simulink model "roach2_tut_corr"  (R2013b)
settings: Solver=VariableStepDiscrete  SolverMode=SingleTasking  StartTime=0.0  StopTime=100  RelTol=1e-3
undefined symbols (not defined in the file): add_latency, addr_width, Bit, bitfield, BitWidth, bram_latency, burst_size, casper_library_scopes, conv_latency, data_width, DelayLen, fan_latency, FFTSize, FFTStage, getfield, increment, led, Location, Lower, mult_latency, mux_latency, n_bits, n_bits_data, n_inputs, n_streams, n_taps, neg_latency, negate_latency, nsamples, pfb_size, pulse_len, reset_period, ROACH, ROACH2, snapshot, sx475t, sync_period, sync_period_bits, Upper, UseCounter, Width
libraries: xbsIndex_r4 x24444, casper_library_misc x73, xbsReplacements_r4 x34, casper_library_delays x14, xps_library x7
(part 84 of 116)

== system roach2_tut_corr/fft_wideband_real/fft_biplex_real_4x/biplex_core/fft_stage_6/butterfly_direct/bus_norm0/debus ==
  bus_in : Inport
  reinterpret{1..16} (16 alike) : xbsIndex_r4/Reinterpret  force_arith_type=on  arith_type="Signed  (2's comp)"  force_bin_pt=on  bin_pt=17  block_type=reinterpret
  slice1 : xbsIndex_r4/Slice  nbits=20  boolean_output=off  mode=Upper Bit Location + Width  bit1=-300  base1=MSB of Input  bit0=0  base0=LSB of Input  dbl_ovrd=off  block_type=slice
  slice10 : xbsIndex_r4/Slice  nbits=20  boolean_output=off  mode=Upper Bit Location + Width  bit1=-120  base1=MSB of Input  bit0=0  base0=LSB of Input  dbl_ovrd=off  block_type=slice
  slice11 : xbsIndex_r4/Slice  nbits=20  boolean_output=off  mode=Upper Bit Location + Width  bit1=-100  base1=MSB of Input  bit0=0  base0=LSB of Input  dbl_ovrd=off  block_type=slice
  slice12 : xbsIndex_r4/Slice  nbits=20  boolean_output=off  mode=Upper Bit Location + Width  bit1=-80  base1=MSB of Input  bit0=0  base0=LSB of Input  dbl_ovrd=off  block_type=slice
  slice13 : xbsIndex_r4/Slice  nbits=20  boolean_output=off  mode=Upper Bit Location + Width  bit1=-60  base1=MSB of Input  bit0=0  base0=LSB of Input  dbl_ovrd=off  block_type=slice
  slice14 : xbsIndex_r4/Slice  nbits=20  boolean_output=off  mode=Upper Bit Location + Width  bit1=-40  base1=MSB of Input  bit0=0  base0=LSB of Input  dbl_ovrd=off  block_type=slice
  slice15 : xbsIndex_r4/Slice  nbits=20  boolean_output=off  mode=Upper Bit Location + Width  bit1=-20  base1=MSB of Input  bit0=0  base0=LSB of Input  dbl_ovrd=off  block_type=slice
  slice16 : xbsIndex_r4/Slice  nbits=20  boolean_output=off  mode=Upper Bit Location + Width  bit1=0  base1=MSB of Input  bit0=0  base0=LSB of Input  dbl_ovrd=off  block_type=slice
  slice2 : xbsIndex_r4/Slice  nbits=20  boolean_output=off  mode=Upper Bit Location + Width  bit1=-280  base1=MSB of Input  bit0=0  base0=LSB of Input  dbl_ovrd=off  block_type=slice
  slice3 : xbsIndex_r4/Slice  nbits=20  boolean_output=off  mode=Upper Bit Location + Width  bit1=-260  base1=MSB of Input  bit0=0  base0=LSB of Input  dbl_ovrd=off  block_type=slice
  slice4 : xbsIndex_r4/Slice  nbits=20  boolean_output=off  mode=Upper Bit Location + Width  bit1=-240  base1=MSB of Input  bit0=0  base0=LSB of Input  dbl_ovrd=off  block_type=slice
  slice5 : xbsIndex_r4/Slice  nbits=20  boolean_output=off  mode=Upper Bit Location + Width  bit1=-220  base1=MSB of Input  bit0=0  base0=LSB of Input  dbl_ovrd=off  block_type=slice
  slice6 : xbsIndex_r4/Slice  nbits=20  boolean_output=off  mode=Upper Bit Location + Width  bit1=-200  base1=MSB of Input  bit0=0  base0=LSB of Input  dbl_ovrd=off  block_type=slice
  slice7 : xbsIndex_r4/Slice  nbits=20  boolean_output=off  mode=Upper Bit Location + Width  bit1=-180  base1=MSB of Input  bit0=0  base0=LSB of Input  dbl_ovrd=off  block_type=slice
  slice8 : xbsIndex_r4/Slice  nbits=20  boolean_output=off  mode=Upper Bit Location + Width  bit1=-160  base1=MSB of Input  bit0=0  base0=LSB of Input  dbl_ovrd=off  block_type=slice
  slice9 : xbsIndex_r4/Slice  nbits=20  boolean_output=off  mode=Upper Bit Location + Width  bit1=-140  base1=MSB of Input  bit0=0  base0=LSB of Input  dbl_ovrd=off  block_type=slice
  msb_out16 : Outport
  out15 : Outport  Port=2
  out14 : Outport  Port=3
  out13 : Outport  Port=4
  out12 : Outport  Port=5
  out11 : Outport  Port=6
  out10 : Outport  Port=7
  out9 : Outport  Port=8
  out8 : Outport  Port=9
  out7 : Outport  Port=10
  out6 : Outport  Port=11
  out5 : Outport  Port=12
  out4 : Outport  Port=13
  out3 : Outport  Port=14
  out2 : Outport  Port=15
  lsb_out1 : Outport  Port=16
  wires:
  bus_in/1 -> slice16/1, slice15/1, slice14/1, slice13/1, slice12/1, slice11/1, slice10/1, slice9/1, slice8/1, slice7/1, slice6/1, slice5/1, slice4/1, slice3/1, slice2/1, slice1/1
  slice16/1 -> reinterpret16/1
  reinterpret16/1 -> msb_out16/1
  slice15/1 -> reinterpret15/1
  reinterpret15/1 -> out15/1
  slice14/1 -> reinterpret14/1
  reinterpret14/1 -> out14/1
  slice13/1 -> reinterpret13/1
  reinterpret13/1 -> out13/1
  slice12/1 -> reinterpret12/1
  reinterpret12/1 -> out12/1
  slice11/1 -> reinterpret11/1
  reinterpret11/1 -> out11/1
  slice10/1 -> reinterpret10/1
  reinterpret10/1 -> out10/1
  slice9/1 -> reinterpret9/1
  reinterpret9/1 -> out9/1
  slice8/1 -> reinterpret8/1
  reinterpret8/1 -> out8/1
  slice7/1 -> reinterpret7/1
  reinterpret7/1 -> out7/1
  slice6/1 -> reinterpret6/1
  reinterpret6/1 -> out6/1
  slice5/1 -> reinterpret5/1
  reinterpret5/1 -> out5/1
  slice4/1 -> reinterpret4/1
  reinterpret4/1 -> out4/1
  slice3/1 -> reinterpret3/1
  reinterpret3/1 -> out3/1
  slice2/1 -> reinterpret2/1
  reinterpret2/1 -> out2/1
  slice1/1 -> reinterpret1/1
  reinterpret1/1 -> lsb_out1/1

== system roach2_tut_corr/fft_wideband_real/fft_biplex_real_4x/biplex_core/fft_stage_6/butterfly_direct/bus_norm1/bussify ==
  in1 : Inport
  in2 : Inport  Port=2
  in3 : Inport  Port=3
  in4 : Inport  Port=4
  in5 : Inport  Port=5
  in6 : Inport  Port=6
  in7 : Inport  Port=7
  in8 : Inport  Port=8
  in9 : Inport  Port=9
  in10 : Inport  Port=10
  in11 : Inport  Port=11
  in12 : Inport  Port=12
  in13 : Inport  Port=13
  in14 : Inport  Port=14
  in15 : Inport  Port=15
  in16 : Inport  Port=16
  concatenate : xbsIndex_r4/Concat  num_inputs=16  dbl_ovrd=off  block_type=concat
  reinterpret{1..16} (16 alike) : xbsIndex_r4/Reinterpret  force_arith_type=on  arith_type=Unsigned  force_bin_pt=on  bin_pt=0  block_type=reinterpret
  bus_out : Outport
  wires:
  concatenate/1 -> bus_out/1
  in1/1 -> reinterpret1/1
  reinterpret1/1 -> concatenate/1
  in2/1 -> reinterpret2/1
  reinterpret2/1 -> concatenate/2
  in3/1 -> reinterpret3/1
  reinterpret3/1 -> concatenate/3
  in4/1 -> reinterpret4/1
  reinterpret4/1 -> concatenate/4
  in5/1 -> reinterpret5/1
  reinterpret5/1 -> concatenate/5
  in6/1 -> reinterpret6/1
  reinterpret6/1 -> concatenate/6
  in7/1 -> reinterpret7/1
  reinterpret7/1 -> concatenate/7
  in8/1 -> reinterpret8/1
  reinterpret8/1 -> concatenate/8
  in9/1 -> reinterpret9/1
  reinterpret9/1 -> concatenate/9
  in10/1 -> reinterpret10/1
  reinterpret10/1 -> concatenate/10
  in11/1 -> reinterpret11/1
  reinterpret11/1 -> concatenate/11
  in12/1 -> reinterpret12/1
  reinterpret12/1 -> concatenate/12
  in13/1 -> reinterpret13/1
  reinterpret13/1 -> concatenate/13
  in14/1 -> reinterpret14/1
  reinterpret14/1 -> concatenate/14
  in15/1 -> reinterpret15/1
  reinterpret15/1 -> concatenate/15
  in16/1 -> reinterpret16/1
  reinterpret16/1 -> concatenate/16

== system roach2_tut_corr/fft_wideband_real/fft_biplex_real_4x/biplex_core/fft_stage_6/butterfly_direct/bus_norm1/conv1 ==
  note: (ones_bit & 1) -> round-to-even (ones_bit ^ 1) -> round-to-odd (sign_bit & 1)-> round-to-zero (sign_bit ^ 1) -> round-to-inf (X ~| 1) -> round half down (X | 1) -> round half up
  in : Inport
  Concat : xbsIndex_r4/Concat  num_inputs=2  dbl_ovrd=off  block_type=concat
  Constant : xbsIndex_r4/Constant  const=1  gui_display_data_type=Fixed-point  arith_type=Unsigned  n_bits=1  bin_pt=0  preci_type=Single  exp_width=8  frac_width=24  explicit_period=off  period=1  equ=P=C  opselect=C  inp2=PCIN>>17  opr=+  inp1=P  carry=CIN  dbl_ovrd=off  block_type=constant
  Reinterpret : xbsIndex_r4/Reinterpret  force_arith_type=on  arith_type=Unsigned  force_bin_pt=on  bin_pt=0  block_type=reinterpret
  adder : xbsIndex_r4/AddSub  mode=Addition  use_carryin=off  use_carryout=off  en=off  latency=0  precision=User Defined  arith_type="Signed  (2's comp)"  n_bits=21  bin_pt=18  quantization=Truncate  overflow=Wrap  dbl_ovrd=off  use_behavioral_HDL=off  hw_selection=Fabric  pipelined=on  use_rpm=on  block_type=addsub
  almost_half : xbsIndex_r4/Constant  const=0  gui_display_data_type=Fixed-point  arith_type=Unsigned  n_bits=19  bin_pt=0  preci_type=Single  exp_width=8  frac_width=24  explicit_period=off  period=1  equ=P=C  opselect=C  inp2=PCIN>>17  opr=+  inp1=P  carry=CIN  dbl_ovrd=off  block_type=constant
  bit : xbsIndex_r4/Slice  nbits=1  boolean_output=off  mode=Lower Bit Location + Width  bit1=0  base1=MSB of Input  bit0=0  base0=LSB of Input  dbl_ovrd=off  block_type=slice
  force1 : xbsIndex_r4/Reinterpret  force_arith_type=on  arith_type="Signed  (2's comp)"  force_bin_pt=on  bin_pt=19  block_type=reinterpret
  force2 : xbsIndex_r4/Reinterpret  force_arith_type=off  arith_type="Signed  (2's comp)"  force_bin_pt=on  bin_pt=19  block_type=reinterpret
  tweak_op : xbsIndex_r4/Logical  logical_function=NOR  inputs=2  en=off  latency=0  precision=Full  arith_type=Unsigned  n_bits=8  bin_pt=2  align_bp=on  dbl_ovrd=off  block_type=logical
  out : Outport
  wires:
  tweak_op/1 -> Concat/2
  Constant/1 -> tweak_op/2
  bit/1 -> tweak_op/1
  almost_half/1 -> force2/1
  in/1 -> Reinterpret/1, bit/1
  Concat/1 -> force1/1
  Reinterpret/1 -> Concat/1
  force1/1 -> adder/1
  force2/1 -> adder/2
  adder/1 -> out/1

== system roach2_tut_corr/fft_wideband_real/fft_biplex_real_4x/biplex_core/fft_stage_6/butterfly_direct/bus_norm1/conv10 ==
  note: (ones_bit & 1) -> round-to-even (ones_bit ^ 1) -> round-to-odd (sign_bit & 1)-> round-to-zero (sign_bit ^ 1) -> round-to-inf (X ~| 1) -> round half down (X | 1) -> round half up
  in : Inport
  Concat : xbsIndex_r4/Concat  num_inputs=2  dbl_ovrd=off  block_type=concat
  Constant : xbsIndex_r4/Constant  const=1  gui_display_data_type=Fixed-point  arith_type=Unsigned  n_bits=1  bin_pt=0  preci_type=Single  exp_width=8  frac_width=24  explicit_period=off  period=1  equ=P=C  opselect=C  inp2=PCIN>>17  opr=+  inp1=P  carry=CIN  dbl_ovrd=off  block_type=constant
  Reinterpret : xbsIndex_r4/Reinterpret  force_arith_type=on  arith_type=Unsigned  force_bin_pt=on  bin_pt=0  block_type=reinterpret
  adder : xbsIndex_r4/AddSub  mode=Addition  use_carryin=off  use_carryout=off  en=off  latency=0  precision=User Defined  arith_type="Signed  (2's comp)"  n_bits=21  bin_pt=18  quantization=Truncate  overflow=Wrap  dbl_ovrd=off  use_behavioral_HDL=off  hw_selection=Fabric  pipelined=on  use_rpm=on  block_type=addsub
  almost_half : xbsIndex_r4/Constant  const=0  gui_display_data_type=Fixed-point  arith_type=Unsigned  n_bits=19  bin_pt=0  preci_type=Single  exp_width=8  frac_width=24  explicit_period=off  period=1  equ=P=C  opselect=C  inp2=PCIN>>17  opr=+  inp1=P  carry=CIN  dbl_ovrd=off  block_type=constant
  bit : xbsIndex_r4/Slice  nbits=1  boolean_output=off  mode=Lower Bit Location + Width  bit1=0  base1=MSB of Input  bit0=0  base0=LSB of Input  dbl_ovrd=off  block_type=slice
  force1 : xbsIndex_r4/Reinterpret  force_arith_type=on  arith_type="Signed  (2's comp)"  force_bin_pt=on  bin_pt=19  block_type=reinterpret
  force2 : xbsIndex_r4/Reinterpret  force_arith_type=off  arith_type="Signed  (2's comp)"  force_bin_pt=on  bin_pt=19  block_type=reinterpret
  tweak_op : xbsIndex_r4/Logical  logical_function=NOR  inputs=2  en=off  latency=0  precision=Full  arith_type=Unsigned  n_bits=8  bin_pt=2  align_bp=on  dbl_ovrd=off  block_type=logical
  out : Outport
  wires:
  tweak_op/1 -> Concat/2
  Constant/1 -> tweak_op/2
  bit/1 -> tweak_op/1
  almost_half/1 -> force2/1
  in/1 -> Reinterpret/1, bit/1
  Concat/1 -> force1/1
  Reinterpret/1 -> Concat/1
  force1/1 -> adder/1
  force2/1 -> adder/2
  adder/1 -> out/1

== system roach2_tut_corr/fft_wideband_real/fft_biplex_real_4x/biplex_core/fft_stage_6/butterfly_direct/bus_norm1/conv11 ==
  note: (ones_bit & 1) -> round-to-even (ones_bit ^ 1) -> round-to-odd (sign_bit & 1)-> round-to-zero (sign_bit ^ 1) -> round-to-inf (X ~| 1) -> round half down (X | 1) -> round half up
  in : Inport
  Concat : xbsIndex_r4/Concat  num_inputs=2  dbl_ovrd=off  block_type=concat
  Constant : xbsIndex_r4/Constant  const=1  gui_display_data_type=Fixed-point  arith_type=Unsigned  n_bits=1  bin_pt=0  preci_type=Single  exp_width=8  frac_width=24  explicit_period=off  period=1  equ=P=C  opselect=C  inp2=PCIN>>17  opr=+  inp1=P  carry=CIN  dbl_ovrd=off  block_type=constant
  Reinterpret : xbsIndex_r4/Reinterpret  force_arith_type=on  arith_type=Unsigned  force_bin_pt=on  bin_pt=0  block_type=reinterpret
  adder : xbsIndex_r4/AddSub  mode=Addition  use_carryin=off  use_carryout=off  en=off  latency=0  precision=User Defined  arith_type="Signed  (2's comp)"  n_bits=21  bin_pt=18  quantization=Truncate  overflow=Wrap  dbl_ovrd=off  use_behavioral_HDL=off  hw_selection=Fabric  pipelined=on  use_rpm=on  block_type=addsub
  almost_half : xbsIndex_r4/Constant  const=0  gui_display_data_type=Fixed-point  arith_type=Unsigned  n_bits=19  bin_pt=0  preci_type=Single  exp_width=8  frac_width=24  explicit_period=off  period=1  equ=P=C  opselect=C  inp2=PCIN>>17  opr=+  inp1=P  carry=CIN  dbl_ovrd=off  block_type=constant
  bit : xbsIndex_r4/Slice  nbits=1  boolean_output=off  mode=Lower Bit Location + Width  bit1=0  base1=MSB of Input  bit0=0  base0=LSB of Input  dbl_ovrd=off  block_type=slice
  force1 : xbsIndex_r4/Reinterpret  force_arith_type=on  arith_type="Signed  (2's comp)"  force_bin_pt=on  bin_pt=19  block_type=reinterpret
  force2 : xbsIndex_r4/Reinterpret  force_arith_type=off  arith_type="Signed  (2's comp)"  force_bin_pt=on  bin_pt=19  block_type=reinterpret
  tweak_op : xbsIndex_r4/Logical  logical_function=NOR  inputs=2  en=off  latency=0  precision=Full  arith_type=Unsigned  n_bits=8  bin_pt=2  align_bp=on  dbl_ovrd=off  block_type=logical
  out : Outport
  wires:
  tweak_op/1 -> Concat/2
  Constant/1 -> tweak_op/2
  bit/1 -> tweak_op/1
  almost_half/1 -> force2/1
  in/1 -> Reinterpret/1, bit/1
  Concat/1 -> force1/1
  Reinterpret/1 -> Concat/1
  force1/1 -> adder/1
  force2/1 -> adder/2
  adder/1 -> out/1

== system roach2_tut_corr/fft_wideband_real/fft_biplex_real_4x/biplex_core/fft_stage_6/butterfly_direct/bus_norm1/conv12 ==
  note: (ones_bit & 1) -> round-to-even (ones_bit ^ 1) -> round-to-odd (sign_bit & 1)-> round-to-zero (sign_bit ^ 1) -> round-to-inf (X ~| 1) -> round half down (X | 1) -> round half up
  in : Inport
  Concat : xbsIndex_r4/Concat  num_inputs=2  dbl_ovrd=off  block_type=concat
  Constant : xbsIndex_r4/Constant  const=1  gui_display_data_type=Fixed-point  arith_type=Unsigned  n_bits=1  bin_pt=0  preci_type=Single  exp_width=8  frac_width=24  explicit_period=off  period=1  equ=P=C  opselect=C  inp2=PCIN>>17  opr=+  inp1=P  carry=CIN  dbl_ovrd=off  block_type=constant
  Reinterpret : xbsIndex_r4/Reinterpret  force_arith_type=on  arith_type=Unsigned  force_bin_pt=on  bin_pt=0  block_type=reinterpret
  adder : xbsIndex_r4/AddSub  mode=Addition  use_carryin=off  use_carryout=off  en=off  latency=0  precision=User Defined  arith_type="Signed  (2's comp)"  n_bits=21  bin_pt=18  quantization=Truncate  overflow=Wrap  dbl_ovrd=off  use_behavioral_HDL=off  hw_selection=Fabric  pipelined=on  use_rpm=on  block_type=addsub
  almost_half : xbsIndex_r4/Constant  const=0  gui_display_data_type=Fixed-point  arith_type=Unsigned  n_bits=19  bin_pt=0  preci_type=Single  exp_width=8  frac_width=24  explicit_period=off  period=1  equ=P=C  opselect=C  inp2=PCIN>>17  opr=+  inp1=P  carry=CIN  dbl_ovrd=off  block_type=constant
  bit : xbsIndex_r4/Slice  nbits=1  boolean_output=off  mode=Lower Bit Location + Width  bit1=0  base1=MSB of Input  bit0=0  base0=LSB of Input  dbl_ovrd=off  block_type=slice
  force1 : xbsIndex_r4/Reinterpret  force_arith_type=on  arith_type="Signed  (2's comp)"  force_bin_pt=on  bin_pt=19  block_type=reinterpret
  force2 : xbsIndex_r4/Reinterpret  force_arith_type=off  arith_type="Signed  (2's comp)"  force_bin_pt=on  bin_pt=19  block_type=reinterpret
  tweak_op : xbsIndex_r4/Logical  logical_function=NOR  inputs=2  en=off  latency=0  precision=Full  arith_type=Unsigned  n_bits=8  bin_pt=2  align_bp=on  dbl_ovrd=off  block_type=logical
  out : Outport
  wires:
  tweak_op/1 -> Concat/2
  Constant/1 -> tweak_op/2
  bit/1 -> tweak_op/1
  almost_half/1 -> force2/1
  in/1 -> Reinterpret/1, bit/1
  Concat/1 -> force1/1
  Reinterpret/1 -> Concat/1
  force1/1 -> adder/1
  force2/1 -> adder/2
  adder/1 -> out/1

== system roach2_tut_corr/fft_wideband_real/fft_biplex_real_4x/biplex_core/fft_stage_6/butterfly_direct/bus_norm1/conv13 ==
  note: (ones_bit & 1) -> round-to-even (ones_bit ^ 1) -> round-to-odd (sign_bit & 1)-> round-to-zero (sign_bit ^ 1) -> round-to-inf (X ~| 1) -> round half down (X | 1) -> round half up
  in : Inport
  Concat : xbsIndex_r4/Concat  num_inputs=2  dbl_ovrd=off  block_type=concat
  Constant : xbsIndex_r4/Constant  const=1  gui_display_data_type=Fixed-point  arith_type=Unsigned  n_bits=1  bin_pt=0  preci_type=Single  exp_width=8  frac_width=24  explicit_period=off  period=1  equ=P=C  opselect=C  inp2=PCIN>>17  opr=+  inp1=P  carry=CIN  dbl_ovrd=off  block_type=constant
  Reinterpret : xbsIndex_r4/Reinterpret  force_arith_type=on  arith_type=Unsigned  force_bin_pt=on  bin_pt=0  block_type=reinterpret
  adder : xbsIndex_r4/AddSub  mode=Addition  use_carryin=off  use_carryout=off  en=off  latency=0  precision=User Defined  arith_type="Signed  (2's comp)"  n_bits=21  bin_pt=18  quantization=Truncate  overflow=Wrap  dbl_ovrd=off  use_behavioral_HDL=off  hw_selection=Fabric  pipelined=on  use_rpm=on  block_type=addsub
  almost_half : xbsIndex_r4/Constant  const=0  gui_display_data_type=Fixed-point  arith_type=Unsigned  n_bits=19  bin_pt=0  preci_type=Single  exp_width=8  frac_width=24  explicit_period=off  period=1  equ=P=C  opselect=C  inp2=PCIN>>17  opr=+  inp1=P  carry=CIN  dbl_ovrd=off  block_type=constant
  bit : xbsIndex_r4/Slice  nbits=1  boolean_output=off  mode=Lower Bit Location + Width  bit1=0  base1=MSB of Input  bit0=0  base0=LSB of Input  dbl_ovrd=off  block_type=slice
  force1 : xbsIndex_r4/Reinterpret  force_arith_type=on  arith_type="Signed  (2's comp)"  force_bin_pt=on  bin_pt=19  block_type=reinterpret
  force2 : xbsIndex_r4/Reinterpret  force_arith_type=off  arith_type="Signed  (2's comp)"  force_bin_pt=on  bin_pt=19  block_type=reinterpret
  tweak_op : xbsIndex_r4/Logical  logical_function=NOR  inputs=2  en=off  latency=0  precision=Full  arith_type=Unsigned  n_bits=8  bin_pt=2  align_bp=on  dbl_ovrd=off  block_type=logical
  out : Outport
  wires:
  tweak_op/1 -> Concat/2
  Constant/1 -> tweak_op/2
  bit/1 -> tweak_op/1
  almost_half/1 -> force2/1
  in/1 -> Reinterpret/1, bit/1
  Concat/1 -> force1/1
  Reinterpret/1 -> Concat/1
  force1/1 -> adder/1
  force2/1 -> adder/2
  adder/1 -> out/1

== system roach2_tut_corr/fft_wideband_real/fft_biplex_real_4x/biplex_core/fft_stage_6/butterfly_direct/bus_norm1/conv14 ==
  note: (ones_bit & 1) -> round-to-even (ones_bit ^ 1) -> round-to-odd (sign_bit & 1)-> round-to-zero (sign_bit ^ 1) -> round-to-inf (X ~| 1) -> round half down (X | 1) -> round half up
  in : Inport
  Concat : xbsIndex_r4/Concat  num_inputs=2  dbl_ovrd=off  block_type=concat
  Constant : xbsIndex_r4/Constant  const=1  gui_display_data_type=Fixed-point  arith_type=Unsigned  n_bits=1  bin_pt=0  preci_type=Single  exp_width=8  frac_width=24  explicit_period=off  period=1  equ=P=C  opselect=C  inp2=PCIN>>17  opr=+  inp1=P  carry=CIN  dbl_ovrd=off  block_type=constant
  Reinterpret : xbsIndex_r4/Reinterpret  force_arith_type=on  arith_type=Unsigned  force_bin_pt=on  bin_pt=0  block_type=reinterpret
  adder : xbsIndex_r4/AddSub  mode=Addition  use_carryin=off  use_carryout=off  en=off  latency=0  precision=User Defined  arith_type="Signed  (2's comp)"  n_bits=21  bin_pt=18  quantization=Truncate  overflow=Wrap  dbl_ovrd=off  use_behavioral_HDL=off  hw_selection=Fabric  pipelined=on  use_rpm=on  block_type=addsub
  almost_half : xbsIndex_r4/Constant  const=0  gui_display_data_type=Fixed-point  arith_type=Unsigned  n_bits=19  bin_pt=0  preci_type=Single  exp_width=8  frac_width=24  explicit_period=off  period=1  equ=P=C  opselect=C  inp2=PCIN>>17  opr=+  inp1=P  carry=CIN  dbl_ovrd=off  block_type=constant
  bit : xbsIndex_r4/Slice  nbits=1  boolean_output=off  mode=Lower Bit Location + Width  bit1=0  base1=MSB of Input  bit0=0  base0=LSB of Input  dbl_ovrd=off  block_type=slice
  force1 : xbsIndex_r4/Reinterpret  force_arith_type=on  arith_type="Signed  (2's comp)"  force_bin_pt=on  bin_pt=19  block_type=reinterpret
  force2 : xbsIndex_r4/Reinterpret  force_arith_type=off  arith_type="Signed  (2's comp)"  force_bin_pt=on  bin_pt=19  block_type=reinterpret
  tweak_op : xbsIndex_r4/Logical  logical_function=NOR  inputs=2  en=off  latency=0  precision=Full  arith_type=Unsigned  n_bits=8  bin_pt=2  align_bp=on  dbl_ovrd=off  block_type=logical
  out : Outport
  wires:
  tweak_op/1 -> Concat/2
  Constant/1 -> tweak_op/2
  bit/1 -> tweak_op/1
  almost_half/1 -> force2/1
  in/1 -> Reinterpret/1, bit/1
  Concat/1 -> force1/1
  Reinterpret/1 -> Concat/1
  force1/1 -> adder/1
  force2/1 -> adder/2
  adder/1 -> out/1

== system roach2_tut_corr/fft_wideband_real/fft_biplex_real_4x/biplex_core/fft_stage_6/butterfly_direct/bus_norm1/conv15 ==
  note: (ones_bit & 1) -> round-to-even (ones_bit ^ 1) -> round-to-odd (sign_bit & 1)-> round-to-zero (sign_bit ^ 1) -> round-to-inf (X ~| 1) -> round half down (X | 1) -> round half up
  in : Inport
  Concat : xbsIndex_r4/Concat  num_inputs=2  dbl_ovrd=off  block_type=concat
  Constant : xbsIndex_r4/Constant  const=1  gui_display_data_type=Fixed-point  arith_type=Unsigned  n_bits=1  bin_pt=0  preci_type=Single  exp_width=8  frac_width=24  explicit_period=off  period=1  equ=P=C  opselect=C  inp2=PCIN>>17  opr=+  inp1=P  carry=CIN  dbl_ovrd=off  block_type=constant
  Reinterpret : xbsIndex_r4/Reinterpret  force_arith_type=on  arith_type=Unsigned  force_bin_pt=on  bin_pt=0  block_type=reinterpret
  adder : xbsIndex_r4/AddSub  mode=Addition  use_carryin=off  use_carryout=off  en=off  latency=0  precision=User Defined  arith_type="Signed  (2's comp)"  n_bits=21  bin_pt=18  quantization=Truncate  overflow=Wrap  dbl_ovrd=off  use_behavioral_HDL=off  hw_selection=Fabric  pipelined=on  use_rpm=on  block_type=addsub
  almost_half : xbsIndex_r4/Constant  const=0  gui_display_data_type=Fixed-point  arith_type=Unsigned  n_bits=19  bin_pt=0  preci_type=Single  exp_width=8  frac_width=24  explicit_period=off  period=1  equ=P=C  opselect=C  inp2=PCIN>>17  opr=+  inp1=P  carry=CIN  dbl_ovrd=off  block_type=constant
  bit : xbsIndex_r4/Slice  nbits=1  boolean_output=off  mode=Lower Bit Location + Width  bit1=0  base1=MSB of Input  bit0=0  base0=LSB of Input  dbl_ovrd=off  block_type=slice
  force1 : xbsIndex_r4/Reinterpret  force_arith_type=on  arith_type="Signed  (2's comp)"  force_bin_pt=on  bin_pt=19  block_type=reinterpret
  force2 : xbsIndex_r4/Reinterpret  force_arith_type=off  arith_type="Signed  (2's comp)"  force_bin_pt=on  bin_pt=19  block_type=reinterpret
  tweak_op : xbsIndex_r4/Logical  logical_function=NOR  inputs=2  en=off  latency=0  precision=Full  arith_type=Unsigned  n_bits=8  bin_pt=2  align_bp=on  dbl_ovrd=off  block_type=logical
  out : Outport
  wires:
  tweak_op/1 -> Concat/2
  Constant/1 -> tweak_op/2
  bit/1 -> tweak_op/1
  almost_half/1 -> force2/1
  in/1 -> Reinterpret/1, bit/1
  Concat/1 -> force1/1
  Reinterpret/1 -> Concat/1
  force1/1 -> adder/1
  force2/1 -> adder/2
  adder/1 -> out/1

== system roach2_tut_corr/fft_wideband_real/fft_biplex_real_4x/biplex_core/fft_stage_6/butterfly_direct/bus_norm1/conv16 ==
  note: (ones_bit & 1) -> round-to-even (ones_bit ^ 1) -> round-to-odd (sign_bit & 1)-> round-to-zero (sign_bit ^ 1) -> round-to-inf (X ~| 1) -> round half down (X | 1) -> round half up
  in : Inport
  Concat : xbsIndex_r4/Concat  num_inputs=2  dbl_ovrd=off  block_type=concat
  Constant : xbsIndex_r4/Constant  const=1  gui_display_data_type=Fixed-point  arith_type=Unsigned  n_bits=1  bin_pt=0  preci_type=Single  exp_width=8  frac_width=24  explicit_period=off  period=1  equ=P=C  opselect=C  inp2=PCIN>>17  opr=+  inp1=P  carry=CIN  dbl_ovrd=off  block_type=constant
  Reinterpret : xbsIndex_r4/Reinterpret  force_arith_type=on  arith_type=Unsigned  force_bin_pt=on  bin_pt=0  block_type=reinterpret
  adder : xbsIndex_r4/AddSub  mode=Addition  use_carryin=off  use_carryout=off  en=off  latency=0  precision=User Defined  arith_type="Signed  (2's comp)"  n_bits=21  bin_pt=18  quantization=Truncate  overflow=Wrap  dbl_ovrd=off  use_behavioral_HDL=off  hw_selection=Fabric  pipelined=on  use_rpm=on  block_type=addsub
  almost_half : xbsIndex_r4/Constant  const=0  gui_display_data_type=Fixed-point  arith_type=Unsigned  n_bits=19  bin_pt=0  preci_type=Single  exp_width=8  frac_width=24  explicit_period=off  period=1  equ=P=C  opselect=C  inp2=PCIN>>17  opr=+  inp1=P  carry=CIN  dbl_ovrd=off  block_type=constant
  bit : xbsIndex_r4/Slice  nbits=1  boolean_output=off  mode=Lower Bit Location + Width  bit1=0  base1=MSB of Input  bit0=0  base0=LSB of Input  dbl_ovrd=off  block_type=slice
  force1 : xbsIndex_r4/Reinterpret  force_arith_type=on  arith_type="Signed  (2's comp)"  force_bin_pt=on  bin_pt=19  block_type=reinterpret
  force2 : xbsIndex_r4/Reinterpret  force_arith_type=off  arith_type="Signed  (2's comp)"  force_bin_pt=on  bin_pt=19  block_type=reinterpret
  tweak_op : xbsIndex_r4/Logical  logical_function=NOR  inputs=2  en=off  latency=0  precision=Full  arith_type=Unsigned  n_bits=8  bin_pt=2  align_bp=on  dbl_ovrd=off  block_type=logical
  out : Outport
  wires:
  tweak_op/1 -> Concat/2
  Constant/1 -> tweak_op/2
  bit/1 -> tweak_op/1
  almost_half/1 -> force2/1
  in/1 -> Reinterpret/1, bit/1
  Concat/1 -> force1/1
  Reinterpret/1 -> Concat/1
  force1/1 -> adder/1
  force2/1 -> adder/2
  adder/1 -> out/1

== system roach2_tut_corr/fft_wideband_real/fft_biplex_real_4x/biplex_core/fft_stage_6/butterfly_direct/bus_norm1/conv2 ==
  note: (ones_bit & 1) -> round-to-even (ones_bit ^ 1) -> round-to-odd (sign_bit & 1)-> round-to-zero (sign_bit ^ 1) -> round-to-inf (X ~| 1) -> round half down (X | 1) -> round half up
  in : Inport
  Concat : xbsIndex_r4/Concat  num_inputs=2  dbl_ovrd=off  block_type=concat
  Constant : xbsIndex_r4/Constant  const=1  gui_display_data_type=Fixed-point  arith_type=Unsigned  n_bits=1  bin_pt=0  preci_type=Single  exp_width=8  frac_width=24  explicit_period=off  period=1  equ=P=C  opselect=C  inp2=PCIN>>17  opr=+  inp1=P  carry=CIN  dbl_ovrd=off  block_type=constant
  Reinterpret : xbsIndex_r4/Reinterpret  force_arith_type=on  arith_type=Unsigned  force_bin_pt=on  bin_pt=0  block_type=reinterpret
  adder : xbsIndex_r4/AddSub  mode=Addition  use_carryin=off  use_carryout=off  en=off  latency=0  precision=User Defined  arith_type="Signed  (2's comp)"  n_bits=21  bin_pt=18  quantization=Truncate  overflow=Wrap  dbl_ovrd=off  use_behavioral_HDL=off  hw_selection=Fabric  pipelined=on  use_rpm=on  block_type=addsub
  almost_half : xbsIndex_r4/Constant  const=0  gui_display_data_type=Fixed-point  arith_type=Unsigned  n_bits=19  bin_pt=0  preci_type=Single  exp_width=8  frac_width=24  explicit_period=off  period=1  equ=P=C  opselect=C  inp2=PCIN>>17  opr=+  inp1=P  carry=CIN  dbl_ovrd=off  block_type=constant
  bit : xbsIndex_r4/Slice  nbits=1  boolean_output=off  mode=Lower Bit Location + Width  bit1=0  base1=MSB of Input  bit0=0  base0=LSB of Input  dbl_ovrd=off  block_type=slice
  force1 : xbsIndex_r4/Reinterpret  force_arith_type=on  arith_type="Signed  (2's comp)"  force_bin_pt=on  bin_pt=19  block_type=reinterpret
  force2 : xbsIndex_r4/Reinterpret  force_arith_type=off  arith_type="Signed  (2's comp)"  force_bin_pt=on  bin_pt=19  block_type=reinterpret
  tweak_op : xbsIndex_r4/Logical  logical_function=NOR  inputs=2  en=off  latency=0  precision=Full  arith_type=Unsigned  n_bits=8  bin_pt=2  align_bp=on  dbl_ovrd=off  block_type=logical
  out : Outport
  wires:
  tweak_op/1 -> Concat/2
  Constant/1 -> tweak_op/2
  bit/1 -> tweak_op/1
  almost_half/1 -> force2/1
  in/1 -> Reinterpret/1, bit/1
  Concat/1 -> force1/1
  Reinterpret/1 -> Concat/1
  force1/1 -> adder/1
  force2/1 -> adder/2
  adder/1 -> out/1

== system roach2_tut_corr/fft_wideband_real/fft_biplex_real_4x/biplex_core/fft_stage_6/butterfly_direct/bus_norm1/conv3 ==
  note: (ones_bit & 1) -> round-to-even (ones_bit ^ 1) -> round-to-odd (sign_bit & 1)-> round-to-zero (sign_bit ^ 1) -> round-to-inf (X ~| 1) -> round half down (X | 1) -> round half up
  in : Inport
  Concat : xbsIndex_r4/Concat  num_inputs=2  dbl_ovrd=off  block_type=concat
  Constant : xbsIndex_r4/Constant  const=1  gui_display_data_type=Fixed-point  arith_type=Unsigned  n_bits=1  bin_pt=0  preci_type=Single  exp_width=8  frac_width=24  explicit_period=off  period=1  equ=P=C  opselect=C  inp2=PCIN>>17  opr=+  inp1=P  carry=CIN  dbl_ovrd=off  block_type=constant
  Reinterpret : xbsIndex_r4/Reinterpret  force_arith_type=on  arith_type=Unsigned  force_bin_pt=on  bin_pt=0  block_type=reinterpret
  adder : xbsIndex_r4/AddSub  mode=Addition  use_carryin=off  use_carryout=off  en=off  latency=0  precision=User Defined  arith_type="Signed  (2's comp)"  n_bits=21  bin_pt=18  quantization=Truncate  overflow=Wrap  dbl_ovrd=off  use_behavioral_HDL=off  hw_selection=Fabric  pipelined=on  use_rpm=on  block_type=addsub
  almost_half : xbsIndex_r4/Constant  const=0  gui_display_data_type=Fixed-point  arith_type=Unsigned  n_bits=19  bin_pt=0  preci_type=Single  exp_width=8  frac_width=24  explicit_period=off  period=1  equ=P=C  opselect=C  inp2=PCIN>>17  opr=+  inp1=P  carry=CIN  dbl_ovrd=off  block_type=constant
  bit : xbsIndex_r4/Slice  nbits=1  boolean_output=off  mode=Lower Bit Location + Width  bit1=0  base1=MSB of Input  bit0=0  base0=LSB of Input  dbl_ovrd=off  block_type=slice
  force1 : xbsIndex_r4/Reinterpret  force_arith_type=on  arith_type="Signed  (2's comp)"  force_bin_pt=on  bin_pt=19  block_type=reinterpret
  force2 : xbsIndex_r4/Reinterpret  force_arith_type=off  arith_type="Signed  (2's comp)"  force_bin_pt=on  bin_pt=19  block_type=reinterpret
  tweak_op : xbsIndex_r4/Logical  logical_function=NOR  inputs=2  en=off  latency=0  precision=Full  arith_type=Unsigned  n_bits=8  bin_pt=2  align_bp=on  dbl_ovrd=off  block_type=logical
  out : Outport
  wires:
  tweak_op/1 -> Concat/2
  Constant/1 -> tweak_op/2
  bit/1 -> tweak_op/1
  almost_half/1 -> force2/1
  in/1 -> Reinterpret/1, bit/1
  Concat/1 -> force1/1
  Reinterpret/1 -> Concat/1
  force1/1 -> adder/1
  force2/1 -> adder/2
  adder/1 -> out/1

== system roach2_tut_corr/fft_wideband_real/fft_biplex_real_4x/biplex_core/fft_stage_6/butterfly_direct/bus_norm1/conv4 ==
  note: (ones_bit & 1) -> round-to-even (ones_bit ^ 1) -> round-to-odd (sign_bit & 1)-> round-to-zero (sign_bit ^ 1) -> round-to-inf (X ~| 1) -> round half down (X | 1) -> round half up
  in : Inport
  Concat : xbsIndex_r4/Concat  num_inputs=2  dbl_ovrd=off  block_type=concat
  Constant : xbsIndex_r4/Constant  const=1  gui_display_data_type=Fixed-point  arith_type=Unsigned  n_bits=1  bin_pt=0  preci_type=Single  exp_width=8  frac_width=24  explicit_period=off  period=1  equ=P=C  opselect=C  inp2=PCIN>>17  opr=+  inp1=P  carry=CIN  dbl_ovrd=off  block_type=constant
  Reinterpret : xbsIndex_r4/Reinterpret  force_arith_type=on  arith_type=Unsigned  force_bin_pt=on  bin_pt=0  block_type=reinterpret
  adder : xbsIndex_r4/AddSub  mode=Addition  use_carryin=off  use_carryout=off  en=off  latency=0  precision=User Defined  arith_type="Signed  (2's comp)"  n_bits=21  bin_pt=18  quantization=Truncate  overflow=Wrap  dbl_ovrd=off  use_behavioral_HDL=off  hw_selection=Fabric  pipelined=on  use_rpm=on  block_type=addsub
  almost_half : xbsIndex_r4/Constant  const=0  gui_display_data_type=Fixed-point  arith_type=Unsigned  n_bits=19  bin_pt=0  preci_type=Single  exp_width=8  frac_width=24  explicit_period=off  period=1  equ=P=C  opselect=C  inp2=PCIN>>17  opr=+  inp1=P  carry=CIN  dbl_ovrd=off  block_type=constant
  bit : xbsIndex_r4/Slice  nbits=1  boolean_output=off  mode=Lower Bit Location + Width  bit1=0  base1=MSB of Input  bit0=0  base0=LSB of Input  dbl_ovrd=off  block_type=slice
  force1 : xbsIndex_r4/Reinterpret  force_arith_type=on  arith_type="Signed  (2's comp)"  force_bin_pt=on  bin_pt=19  block_type=reinterpret
  force2 : xbsIndex_r4/Reinterpret  force_arith_type=off  arith_type="Signed  (2's comp)"  force_bin_pt=on  bin_pt=19  block_type=reinterpret
  tweak_op : xbsIndex_r4/Logical  logical_function=NOR  inputs=2  en=off  latency=0  precision=Full  arith_type=Unsigned  n_bits=8  bin_pt=2  align_bp=on  dbl_ovrd=off  block_type=logical
  out : Outport
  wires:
  tweak_op/1 -> Concat/2
  Constant/1 -> tweak_op/2
  bit/1 -> tweak_op/1
  almost_half/1 -> force2/1
  in/1 -> Reinterpret/1, bit/1
  Concat/1 -> force1/1
  Reinterpret/1 -> Concat/1
  force1/1 -> adder/1
  force2/1 -> adder/2
  adder/1 -> out/1

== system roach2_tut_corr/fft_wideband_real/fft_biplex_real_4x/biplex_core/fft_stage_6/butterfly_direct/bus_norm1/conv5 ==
  note: (ones_bit & 1) -> round-to-even (ones_bit ^ 1) -> round-to-odd (sign_bit & 1)-> round-to-zero (sign_bit ^ 1) -> round-to-inf (X ~| 1) -> round half down (X | 1) -> round half up
  in : Inport
  Concat : xbsIndex_r4/Concat  num_inputs=2  dbl_ovrd=off  block_type=concat
  Constant : xbsIndex_r4/Constant  const=1  gui_display_data_type=Fixed-point  arith_type=Unsigned  n_bits=1  bin_pt=0  preci_type=Single  exp_width=8  frac_width=24  explicit_period=off  period=1  equ=P=C  opselect=C  inp2=PCIN>>17  opr=+  inp1=P  carry=CIN  dbl_ovrd=off  block_type=constant
  Reinterpret : xbsIndex_r4/Reinterpret  force_arith_type=on  arith_type=Unsigned  force_bin_pt=on  bin_pt=0  block_type=reinterpret
  adder : xbsIndex_r4/AddSub  mode=Addition  use_carryin=off  use_carryout=off  en=off  latency=0  precision=User Defined  arith_type="Signed  (2's comp)"  n_bits=21  bin_pt=18  quantization=Truncate  overflow=Wrap  dbl_ovrd=off  use_behavioral_HDL=off  hw_selection=Fabric  pipelined=on  use_rpm=on  block_type=addsub
  almost_half : xbsIndex_r4/Constant  const=0  gui_display_data_type=Fixed-point  arith_type=Unsigned  n_bits=19  bin_pt=0  preci_type=Single  exp_width=8  frac_width=24  explicit_period=off  period=1  equ=P=C  opselect=C  inp2=PCIN>>17  opr=+  inp1=P  carry=CIN  dbl_ovrd=off  block_type=constant
  bit : xbsIndex_r4/Slice  nbits=1  boolean_output=off  mode=Lower Bit Location + Width  bit1=0  base1=MSB of Input  bit0=0  base0=LSB of Input  dbl_ovrd=off  block_type=slice
  force1 : xbsIndex_r4/Reinterpret  force_arith_type=on  arith_type="Signed  (2's comp)"  force_bin_pt=on  bin_pt=19  block_type=reinterpret
  force2 : xbsIndex_r4/Reinterpret  force_arith_type=off  arith_type="Signed  (2's comp)"  force_bin_pt=on  bin_pt=19  block_type=reinterpret
  tweak_op : xbsIndex_r4/Logical  logical_function=NOR  inputs=2  en=off  latency=0  precision=Full  arith_type=Unsigned  n_bits=8  bin_pt=2  align_bp=on  dbl_ovrd=off  block_type=logical
  out : Outport
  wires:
  tweak_op/1 -> Concat/2
  Constant/1 -> tweak_op/2
  bit/1 -> tweak_op/1
  almost_half/1 -> force2/1
  in/1 -> Reinterpret/1, bit/1
  Concat/1 -> force1/1
  Reinterpret/1 -> Concat/1
  force1/1 -> adder/1
  force2/1 -> adder/2
  adder/1 -> out/1

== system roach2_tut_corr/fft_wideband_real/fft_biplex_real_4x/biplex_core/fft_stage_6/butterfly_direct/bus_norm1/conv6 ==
  note: (ones_bit & 1) -> round-to-even (ones_bit ^ 1) -> round-to-odd (sign_bit & 1)-> round-to-zero (sign_bit ^ 1) -> round-to-inf (X ~| 1) -> round half down (X | 1) -> round half up
  in : Inport
  Concat : xbsIndex_r4/Concat  num_inputs=2  dbl_ovrd=off  block_type=concat
  Constant : xbsIndex_r4/Constant  const=1  gui_display_data_type=Fixed-point  arith_type=Unsigned  n_bits=1  bin_pt=0  preci_type=Single  exp_width=8  frac_width=24  explicit_period=off  period=1  equ=P=C  opselect=C  inp2=PCIN>>17  opr=+  inp1=P  carry=CIN  dbl_ovrd=off  block_type=constant
  Reinterpret : xbsIndex_r4/Reinterpret  force_arith_type=on  arith_type=Unsigned  force_bin_pt=on  bin_pt=0  block_type=reinterpret
  adder : xbsIndex_r4/AddSub  mode=Addition  use_carryin=off  use_carryout=off  en=off  latency=0  precision=User Defined  arith_type="Signed  (2's comp)"  n_bits=21  bin_pt=18  quantization=Truncate  overflow=Wrap  dbl_ovrd=off  use_behavioral_HDL=off  hw_selection=Fabric  pipelined=on  use_rpm=on  block_type=addsub
  almost_half : xbsIndex_r4/Constant  const=0  gui_display_data_type=Fixed-point  arith_type=Unsigned  n_bits=19  bin_pt=0  preci_type=Single  exp_width=8  frac_width=24  explicit_period=off  period=1  equ=P=C  opselect=C  inp2=PCIN>>17  opr=+  inp1=P  carry=CIN  dbl_ovrd=off  block_type=constant
  bit : xbsIndex_r4/Slice  nbits=1  boolean_output=off  mode=Lower Bit Location + Width  bit1=0  base1=MSB of Input  bit0=0  base0=LSB of Input  dbl_ovrd=off  block_type=slice
  force1 : xbsIndex_r4/Reinterpret  force_arith_type=on  arith_type="Signed  (2's comp)"  force_bin_pt=on  bin_pt=19  block_type=reinterpret
  force2 : xbsIndex_r4/Reinterpret  force_arith_type=off  arith_type="Signed  (2's comp)"  force_bin_pt=on  bin_pt=19  block_type=reinterpret
  tweak_op : xbsIndex_r4/Logical  logical_function=NOR  inputs=2  en=off  latency=0  precision=Full  arith_type=Unsigned  n_bits=8  bin_pt=2  align_bp=on  dbl_ovrd=off  block_type=logical
  out : Outport
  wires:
  tweak_op/1 -> Concat/2
  Constant/1 -> tweak_op/2
  bit/1 -> tweak_op/1
  almost_half/1 -> force2/1
  in/1 -> Reinterpret/1, bit/1
  Concat/1 -> force1/1
  Reinterpret/1 -> Concat/1
  force1/1 -> adder/1
  force2/1 -> adder/2
  adder/1 -> out/1

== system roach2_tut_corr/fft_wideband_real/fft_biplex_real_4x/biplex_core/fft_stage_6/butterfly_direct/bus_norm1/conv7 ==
  note: (ones_bit & 1) -> round-to-even (ones_bit ^ 1) -> round-to-odd (sign_bit & 1)-> round-to-zero (sign_bit ^ 1) -> round-to-inf (X ~| 1) -> round half down (X | 1) -> round half up
  in : Inport
  Concat : xbsIndex_r4/Concat  num_inputs=2  dbl_ovrd=off  block_type=concat
  Constant : xbsIndex_r4/Constant  const=1  gui_display_data_type=Fixed-point  arith_type=Unsigned  n_bits=1  bin_pt=0  preci_type=Single  exp_width=8  frac_width=24  explicit_period=off  period=1  equ=P=C  opselect=C  inp2=PCIN>>17  opr=+  inp1=P  carry=CIN  dbl_ovrd=off  block_type=constant
  Reinterpret : xbsIndex_r4/Reinterpret  force_arith_type=on  arith_type=Unsigned  force_bin_pt=on  bin_pt=0  block_type=reinterpret
  adder : xbsIndex_r4/AddSub  mode=Addition  use_carryin=off  use_carryout=off  en=off  latency=0  precision=User Defined  arith_type="Signed  (2's comp)"  n_bits=21  bin_pt=18  quantization=Truncate  overflow=Wrap  dbl_ovrd=off  use_behavioral_HDL=off  hw_selection=Fabric  pipelined=on  use_rpm=on  block_type=addsub
  almost_half : xbsIndex_r4/Constant  const=0  gui_display_data_type=Fixed-point  arith_type=Unsigned  n_bits=19  bin_pt=0  preci_type=Single  exp_width=8  frac_width=24  explicit_period=off  period=1  equ=P=C  opselect=C  inp2=PCIN>>17  opr=+  inp1=P  carry=CIN  dbl_ovrd=off  block_type=constant
  bit : xbsIndex_r4/Slice  nbits=1  boolean_output=off  mode=Lower Bit Location + Width  bit1=0  base1=MSB of Input  bit0=0  base0=LSB of Input  dbl_ovrd=off  block_type=slice
  force1 : xbsIndex_r4/Reinterpret  force_arith_type=on  arith_type="Signed  (2's comp)"  force_bin_pt=on  bin_pt=19  block_type=reinterpret
  force2 : xbsIndex_r4/Reinterpret  force_arith_type=off  arith_type="Signed  (2's comp)"  force_bin_pt=on  bin_pt=19  block_type=reinterpret
  tweak_op : xbsIndex_r4/Logical  logical_function=NOR  inputs=2  en=off  latency=0  precision=Full  arith_type=Unsigned  n_bits=8  bin_pt=2  align_bp=on  dbl_ovrd=off  block_type=logical
  out : Outport
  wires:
  tweak_op/1 -> Concat/2
  Constant/1 -> tweak_op/2
  bit/1 -> tweak_op/1
  almost_half/1 -> force2/1
  in/1 -> Reinterpret/1, bit/1
  Concat/1 -> force1/1
  Reinterpret/1 -> Concat/1
  force1/1 -> adder/1
  force2/1 -> adder/2
  adder/1 -> out/1

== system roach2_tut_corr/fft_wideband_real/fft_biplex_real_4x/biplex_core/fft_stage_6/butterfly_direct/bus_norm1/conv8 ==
  note: (ones_bit & 1) -> round-to-even (ones_bit ^ 1) -> round-to-odd (sign_bit & 1)-> round-to-zero (sign_bit ^ 1) -> round-to-inf (X ~| 1) -> round half down (X | 1) -> round half up
  in : Inport
  Concat : xbsIndex_r4/Concat  num_inputs=2  dbl_ovrd=off  block_type=concat
  Constant : xbsIndex_r4/Constant  const=1  gui_display_data_type=Fixed-point  arith_type=Unsigned  n_bits=1  bin_pt=0  preci_type=Single  exp_width=8  frac_width=24  explicit_period=off  period=1  equ=P=C  opselect=C  inp2=PCIN>>17  opr=+  inp1=P  carry=CIN  dbl_ovrd=off  block_type=constant
  Reinterpret : xbsIndex_r4/Reinterpret  force_arith_type=on  arith_type=Unsigned  force_bin_pt=on  bin_pt=0  block_type=reinterpret
  adder : xbsIndex_r4/AddSub  mode=Addition  use_carryin=off  use_carryout=off  en=off  latency=0  precision=User Defined  arith_type="Signed  (2's comp)"  n_bits=21  bin_pt=18  quantization=Truncate  overflow=Wrap  dbl_ovrd=off  use_behavioral_HDL=off  hw_selection=Fabric  pipelined=on  use_rpm=on  block_type=addsub
  almost_half : xbsIndex_r4/Constant  const=0  gui_display_data_type=Fixed-point  arith_type=Unsigned  n_bits=19  bin_pt=0  preci_type=Single  exp_width=8  frac_width=24  explicit_period=off  period=1  equ=P=C  opselect=C  inp2=PCIN>>17  opr=+  inp1=P  carry=CIN  dbl_ovrd=off  block_type=constant
  bit : xbsIndex_r4/Slice  nbits=1  boolean_output=off  mode=Lower Bit Location + Width  bit1=0  base1=MSB of Input  bit0=0  base0=LSB of Input  dbl_ovrd=off  block_type=slice
  force1 : xbsIndex_r4/Reinterpret  force_arith_type=on  arith_type="Signed  (2's comp)"  force_bin_pt=on  bin_pt=19  block_type=reinterpret
  force2 : xbsIndex_r4/Reinterpret  force_arith_type=off  arith_type="Signed  (2's comp)"  force_bin_pt=on  bin_pt=19  block_type=reinterpret
  tweak_op : xbsIndex_r4/Logical  logical_function=NOR  inputs=2  en=off  latency=0  precision=Full  arith_type=Unsigned  n_bits=8  bin_pt=2  align_bp=on  dbl_ovrd=off  block_type=logical
  out : Outport
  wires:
  tweak_op/1 -> Concat/2
  Constant/1 -> tweak_op/2
  bit/1 -> tweak_op/1
  almost_half/1 -> force2/1
  in/1 -> Reinterpret/1, bit/1
  Concat/1 -> force1/1
  Reinterpret/1 -> Concat/1
  force1/1 -> adder/1
  force2/1 -> adder/2
  adder/1 -> out/1

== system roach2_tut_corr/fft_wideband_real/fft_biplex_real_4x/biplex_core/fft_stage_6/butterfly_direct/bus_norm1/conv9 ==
  note: (ones_bit & 1) -> round-to-even (ones_bit ^ 1) -> round-to-odd (sign_bit & 1)-> round-to-zero (sign_bit ^ 1) -> round-to-inf (X ~| 1) -> round half down (X | 1) -> round half up
  in : Inport
  Concat : xbsIndex_r4/Concat  num_inputs=2  dbl_ovrd=off  block_type=concat
  Constant : xbsIndex_r4/Constant  const=1  gui_display_data_type=Fixed-point  arith_type=Unsigned  n_bits=1  bin_pt=0  preci_type=Single  exp_width=8  frac_width=24  explicit_period=off  period=1  equ=P=C  opselect=C  inp2=PCIN>>17  opr=+  inp1=P  carry=CIN  dbl_ovrd=off  block_type=constant
  Reinterpret : xbsIndex_r4/Reinterpret  force_arith_type=on  arith_type=Unsigned  force_bin_pt=on  bin_pt=0  block_type=reinterpret
  adder : xbsIndex_r4/AddSub  mode=Addition  use_carryin=off  use_carryout=off  en=off  latency=0  precision=User Defined  arith_type="Signed  (2's comp)"  n_bits=21  bin_pt=18  quantization=Truncate  overflow=Wrap  dbl_ovrd=off  use_behavioral_HDL=off  hw_selection=Fabric  pipelined=on  use_rpm=on  block_type=addsub
  almost_half : xbsIndex_r4/Constant  const=0  gui_display_data_type=Fixed-point  arith_type=Unsigned  n_bits=19  bin_pt=0  preci_type=Single  exp_width=8  frac_width=24  explicit_period=off  period=1  equ=P=C  opselect=C  inp2=PCIN>>17  opr=+  inp1=P  carry=CIN  dbl_ovrd=off  block_type=constant
  bit : xbsIndex_r4/Slice  nbits=1  boolean_output=off  mode=Lower Bit Location + Width  bit1=0  base1=MSB of Input  bit0=0  base0=LSB of Input  dbl_ovrd=off  block_type=slice
  force1 : xbsIndex_r4/Reinterpret  force_arith_type=on  arith_type="Signed  (2's comp)"  force_bin_pt=on  bin_pt=19  block_type=reinterpret
  force2 : xbsIndex_r4/Reinterpret  force_arith_type=off  arith_type="Signed  (2's comp)"  force_bin_pt=on  bin_pt=19  block_type=reinterpret
  tweak_op : xbsIndex_r4/Logical  logical_function=NOR  inputs=2  en=off  latency=0  precision=Full  arith_type=Unsigned  n_bits=8  bin_pt=2  align_bp=on  dbl_ovrd=off  block_type=logical
  out : Outport
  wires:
  tweak_op/1 -> Concat/2
  Constant/1 -> tweak_op/2
  bit/1 -> tweak_op/1
  almost_half/1 -> force2/1
  in/1 -> Reinterpret/1, bit/1
  Concat/1 -> force1/1
  Reinterpret/1 -> Concat/1
  force1/1 -> adder/1
  force2/1 -> adder/2
  adder/1 -> out/1

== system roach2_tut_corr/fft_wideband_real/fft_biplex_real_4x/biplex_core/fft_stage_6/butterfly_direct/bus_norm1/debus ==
  bus_in : Inport
  reinterpret{1..16} (16 alike) : xbsIndex_r4/Reinterpret  force_arith_type=on  arith_type="Signed  (2's comp)"  force_bin_pt=on  bin_pt=18  block_type=reinterpret
  slice1 : xbsIndex_r4/Slice  nbits=20  boolean_output=off  mode=Upper Bit Location + Width  bit1=-300  base1=MSB of Input  bit0=0  base0=LSB of Input  dbl_ovrd=off  block_type=slice
  slice10 : xbsIndex_r4/Slice  nbits=20  boolean_output=off  mode=Upper Bit Location + Width  bit1=-120  base1=MSB of Input  bit0=0  base0=LSB of Input  dbl_ovrd=off  block_type=slice
  slice11 : xbsIndex_r4/Slice  nbits=20  boolean_output=off  mode=Upper Bit Location + Width  bit1=-100  base1=MSB of Input  bit0=0  base0=LSB of Input  dbl_ovrd=off  block_type=slice
  slice12 : xbsIndex_r4/Slice  nbits=20  boolean_output=off  mode=Upper Bit Location + Width  bit1=-80  base1=MSB of Input  bit0=0  base0=LSB of Input  dbl_ovrd=off  block_type=slice
  slice13 : xbsIndex_r4/Slice  nbits=20  boolean_output=off  mode=Upper Bit Location + Width  bit1=-60  base1=MSB of Input  bit0=0  base0=LSB of Input  dbl_ovrd=off  block_type=slice
  slice14 : xbsIndex_r4/Slice  nbits=20  boolean_output=off  mode=Upper Bit Location + Width  bit1=-40  base1=MSB of Input  bit0=0  base0=LSB of Input  dbl_ovrd=off  block_type=slice
  slice15 : xbsIndex_r4/Slice  nbits=20  boolean_output=off  mode=Upper Bit Location + Width  bit1=-20  base1=MSB of Input  bit0=0  base0=LSB of Input  dbl_ovrd=off  block_type=slice
  slice16 : xbsIndex_r4/Slice  nbits=20  boolean_output=off  mode=Upper Bit Location + Width  bit1=0  base1=MSB of Input  bit0=0  base0=LSB of Input  dbl_ovrd=off  block_type=slice
  slice2 : xbsIndex_r4/Slice  nbits=20  boolean_output=off  mode=Upper Bit Location + Width  bit1=-280  base1=MSB of Input  bit0=0  base0=LSB of Input  dbl_ovrd=off  block_type=slice
  slice3 : xbsIndex_r4/Slice  nbits=20  boolean_output=off  mode=Upper Bit Location + Width  bit1=-260  base1=MSB of Input  bit0=0  base0=LSB of Input  dbl_ovrd=off  block_type=slice
  slice4 : xbsIndex_r4/Slice  nbits=20  boolean_output=off  mode=Upper Bit Location + Width  bit1=-240  base1=MSB of Input  bit0=0  base0=LSB of Input  dbl_ovrd=off  block_type=slice
  slice5 : xbsIndex_r4/Slice  nbits=20  boolean_output=off  mode=Upper Bit Location + Width  bit1=-220  base1=MSB of Input  bit0=0  base0=LSB of Input  dbl_ovrd=off  block_type=slice
  slice6 : xbsIndex_r4/Slice  nbits=20  boolean_output=off  mode=Upper Bit Location + Width  bit1=-200  base1=MSB of Input  bit0=0  base0=LSB of Input  dbl_ovrd=off  block_type=slice
  slice7 : xbsIndex_r4/Slice  nbits=20  boolean_output=off  mode=Upper Bit Location + Width  bit1=-180  base1=MSB of Input  bit0=0  base0=LSB of Input  dbl_ovrd=off  block_type=slice
  slice8 : xbsIndex_r4/Slice  nbits=20  boolean_output=off  mode=Upper Bit Location + Width  bit1=-160  base1=MSB of Input  bit0=0  base0=LSB of Input  dbl_ovrd=off  block_type=slice
  slice9 : xbsIndex_r4/Slice  nbits=20  boolean_output=off  mode=Upper Bit Location + Width  bit1=-140  base1=MSB of Input  bit0=0  base0=LSB of Input  dbl_ovrd=off  block_type=slice
  msb_out16 : Outport
  out15 : Outport  Port=2
  out14 : Outport  Port=3
  out13 : Outport  Port=4
  out12 : Outport  Port=5
  out11 : Outport  Port=6
  out10 : Outport  Port=7
  out9 : Outport  Port=8
  out8 : Outport  Port=9
  out7 : Outport  Port=10
  out6 : Outport  Port=11
  out5 : Outport  Port=12
  out4 : Outport  Port=13
  out3 : Outport  Port=14
  out2 : Outport  Port=15
  lsb_out1 : Outport  Port=16
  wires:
  bus_in/1 -> slice16/1, slice15/1, slice14/1, slice13/1, slice12/1, slice11/1, slice10/1, slice9/1, slice8/1, slice7/1, slice6/1, slice5/1, slice4/1, slice3/1, slice2/1, slice1/1
  slice16/1 -> reinterpret16/1
  reinterpret16/1 -> msb_out16/1
  slice15/1 -> reinterpret15/1
  reinterpret15/1 -> out15/1
  slice14/1 -> reinterpret14/1
  reinterpret14/1 -> out14/1
  slice13/1 -> reinterpret13/1
  reinterpret13/1 -> out13/1
  slice12/1 -> reinterpret12/1
  reinterpret12/1 -> out12/1
  slice11/1 -> reinterpret11/1
  reinterpret11/1 -> out11/1
  slice10/1 -> reinterpret10/1
  reinterpret10/1 -> out10/1
  slice9/1 -> reinterpret9/1
  reinterpret9/1 -> out9/1
  slice8/1 -> reinterpret8/1
  reinterpret8/1 -> out8/1
  slice7/1 -> reinterpret7/1
  reinterpret7/1 -> out7/1
  slice6/1 -> reinterpret6/1
  reinterpret6/1 -> out6/1
  slice5/1 -> reinterpret5/1
  reinterpret5/1 -> out5/1
  slice4/1 -> reinterpret4/1
  reinterpret4/1 -> out4/1
  slice3/1 -> reinterpret3/1
  reinterpret3/1 -> out3/1
  slice2/1 -> reinterpret2/1
  reinterpret2/1 -> out2/1
  slice1/1 -> reinterpret1/1
  reinterpret1/1 -> lsb_out1/1
